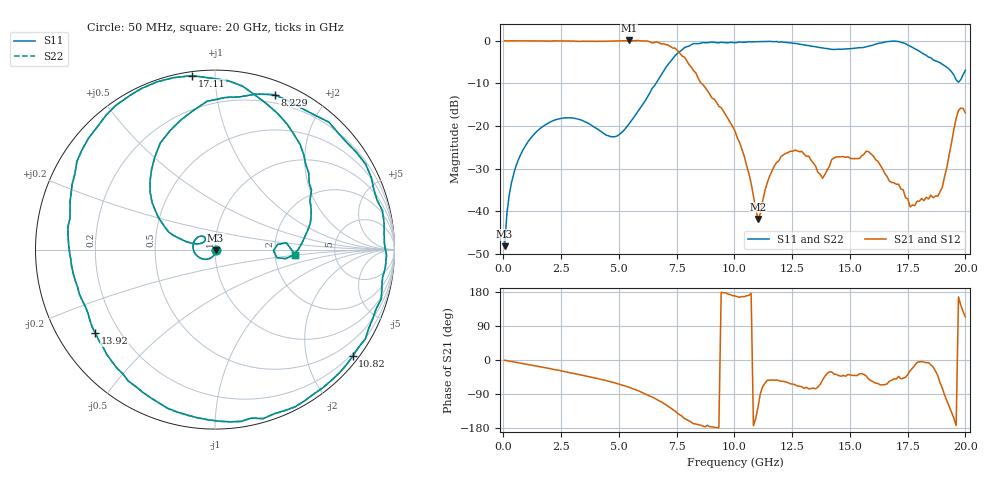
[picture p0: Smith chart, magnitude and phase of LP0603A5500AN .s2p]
!	AVX THIN FILM OPERATION
!	0603 SIZE LOW PASS FILTER P/N LP0603N5500ANTR
!	Created August 2007
!	Network Analyzer HP8720E S.07.64: Feb23, 2000 Serial No.US39172382
#	mhz	S	db	R	50
!	S11	S11	S21	S21	S12	S12	S22	S22
!	dB	Phase	dB	Phase	dB	Phase	dB	Phase
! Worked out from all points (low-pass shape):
!   201 points, 50 MHz to 20 GHz, reference 50 ohm
!   highest |S21| = 0.06 dB at 5.436 GHz (marker M1); lowest = -41.8 dB at 11.02 GHz (marker M2)
!   |S21| within 3 dB of the highest: start of sweep to 7.639 GHz
!   lowest |S11| = -48.2 dB at 50 MHz (marker M3), VSWR 1.01, Z = 50.3 - j0.271 ohm
!   |S11| at or under -10 dB: start of sweep to 6.602 GHz
!   |S22| runs from -48.2 to -0.1 dB; largest |S21 - S12| = 0
!   S11 on the Smith chart (normalised r, x): 50 MHz: 1.01, -0.01; 8.229 GHz: 0.12, +1.45; 10.82 GHz: 0.14, -2.92; 13.92 GHz: 0.11, -0.31; 17.11 GHz: 0.02, +0.88; 20 GHz: 2.61, -0.19
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50  -48.19 -43.7  -0.01 -0.7  -0.01 -0.7  -48.19 -43.7
349.25  -33.26 -91.1  -0.02 -3.8  -0.02 -3.8  -33.26 -91.1
1047.5  -23.81 -125.8  -0.03 -11.8  -0.03 -11.8  -23.81 -125.8
3441.5  -18.78 141.2  -0.11 -40.7  -0.11 -40.7  -18.78 141.2
5436.5  -19.51 162.4  0.06 -71.9  0.06 -71.9  -19.51 162.4
6733.25  -8.82 150.5  -0.47 -107.5  -0.47 -107.5  -8.82 150.5
7431.5  -3.51 117.2  -1.73 -134.9  -1.73 -134.9  -3.51 117.2
8229.5  -0.68 69.0  -7.00 -168.2  -7.00 -168.2  -0.68 69.0
9027.5  -0.31 29.6  -13.45 -176.4  -13.45 -176.4  -0.31 29.6
10025  -0.48 -9.3  -21.21 168.9  -21.21 168.9  -0.48 -9.3
10823  -0.26 -37.8  -36.48 -173.1  -36.48 -173.1  -0.26 -37.8
11022.5  -0.21 -44.8  -41.80 -124.0  -41.80 -124.0  -0.21 -44.8
12020  -0.28 -81.4  -27.15 -56.0  -27.15 -56.0  -0.28 -81.4
13416.5  -1.34 -129.6  -28.68 -74.0  -28.68 -74.0  -1.34 -129.6
13915.25  -1.79 -145.1  -31.42 -43.1  -31.42 -43.1  -1.79 -145.1
15710.75  -1.41 161.9  -25.90 -42.4  -25.90 -42.4  -1.41 161.9
16708.25  -0.17 118.8  -32.91 -55.7  -32.91 -55.7  -0.17 118.8
17107.25  -0.20 97.5  -33.68 -43.5  -33.68 -43.5  -0.20 97.5
17805.5  -1.86 60.2  -38.69 -13.9  -38.69 -13.9  -1.86 60.2
18803  -4.92 19.5  -36.44 -40.9  -36.44 -40.9  -4.92 19.5
19700.75  -9.73 -1.1  -16.35 166.4  -16.35 166.4  -9.73 -1.1
20000  -6.96 -3.8  -16.93 113.5  -16.93 113.5  -6.96 -3.8
